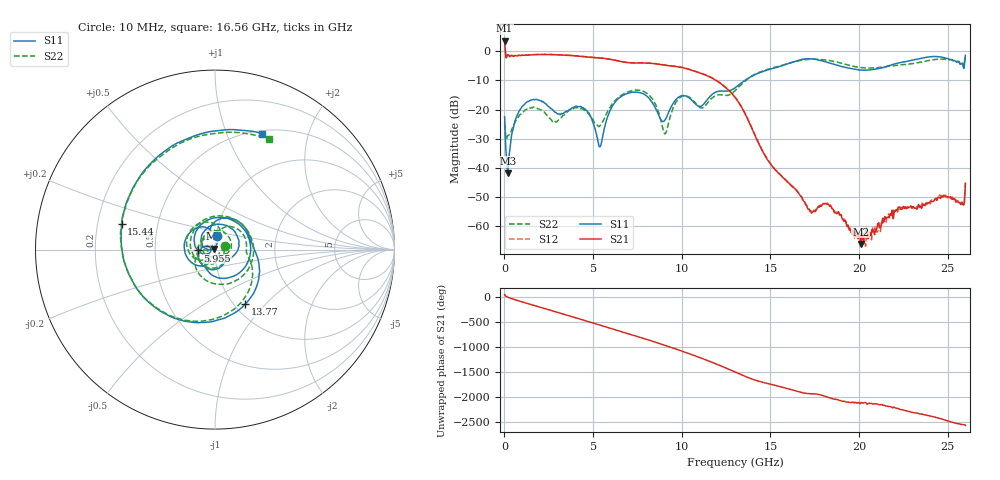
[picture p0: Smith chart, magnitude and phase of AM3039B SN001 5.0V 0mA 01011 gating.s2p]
!Agilent Technologies,E8364B,MY43040894,A.07.50.67
!Agilent E8364B: A.07.50.67
!Date: Tuesday, June 28, 2016 08:05:51
!Correction: S11(Full 2 Port(1,2))
!S21(Full 2 Port(1,2))
!S12(Full 2 Port(1,2))
!S22(Full 2 Port(1,2))
!S2P File: Measurements: S11, S21, S12, S22:
# Hz S  dB  R 50
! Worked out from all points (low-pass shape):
!   1601 points, 10 MHz to 26 GHz, reference 50 ohm
!   highest |S21| = 3.66 dB at 10 MHz (marker M1); lowest = -66.2 dB at 20.1 GHz (marker M2)
!   |S21| within 3 dB of the highest: start of sweep to 44.22 MHz
!   lowest |S11| = -41.8 dB at 188.7 MHz (marker M3), VSWR 1.02, Z = 49.4 + j0.587 ohm
!   |S11| at or under -10 dB: start of sweep to 13.56 GHz
!   |S22| runs from -30.2 to -0.9 dB; largest |S21 - S12| = 0.025
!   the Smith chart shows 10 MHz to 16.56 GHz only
!   S11 on the Smith chart (normalised r, x): 10 MHz: 1.01, +0.15; 5.955 GHz: 0.82, -0.01; 13.77 GHz: 1.13, -0.77; 15.44 GHz: 0.30, +0.12; 16.56 GHz: 0.54, +1.35
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1e7  -22.44 82.0  3.66 40.7  3.73 41.6  -24.84 19.6
1.886812e8  -41.84 132.8  -1.25 -10.7  -1.19 -10.6  -28.95 -62.9
1.618131e9  -16.55 64.8  -1.17 -170.2  -1.12 -170.1  -19.18 70.9
2.641488e9  -19.77 -24.1  -1.13 83.5  -1.07 83.7  -23.57 -20.2
3.469919e9  -20.69 -57.0  -1.35 -2.9  -1.30 -2.8  -21.20 -57.1
4.347081e9  -19.18 -132.6  -1.76 -95.4  -1.73 -95.2  -19.70 -158.1
5.955212e9  -20.31 -177.4  -2.76 92.1  -2.68 92.4  -19.31 -146.9
7.612075e9  -14.16 -18.9  -4.01 -82.8  -3.95 -82.4  -13.34 -33.6
8.684162e9  -21.76 -129.3  -4.44 155.0  -4.37 155.4  -20.68 -169.6
9.918688e9  -15.44 -177.5  -5.45 8.9  -5.37 9.4  -15.77 167.2
1.3005e10  -12.54 -8.5  -15.82 -57.3  -15.67 -56.9  -13.54 -19.1
1.376846e10  -9.19 -60.8  -23.92 -172.5  -23.74 -172.2  -9.28 -70.0
1.544156e10  -5.36 164.8  -41.80 21.3  -41.71 20.8  -5.18 155.5
1.656238e10  -3.13 67.8  -48.54 -85.6  -48.42 -85.7  -3.31 64.0
1.734208e10  -2.59 -9.1  -55.55 -128.3  -55.01 -129.0  -2.73 -4.2
1.838168e10  -4.10 -105.7  -53.15 144.7  -52.74 144.1  -3.24 -94.9
2.010352e10  -6.39 122.3  -66.19 47.2  -64.77 44.0  -5.57 132.6
2.167916e10  -4.92 16.5  -57.14 -24.0  -55.79 -22.8  -5.16 22.7
2.31411e10  -2.88 -93.2  -53.88 -149.6  -53.44 -149.5  -4.07 -83.2
2.422943e10  -1.79 178.3  -51.40 130.0  -50.90 126.4  -2.85 -166.0
2.523654e10  -2.91 91.7  -50.81 27.2  -50.07 27.4  -2.94 109.2
2.6e10  -1.52 -21.2  -45.35 -40.0  -45.14 -41.3  -0.92 8.8
